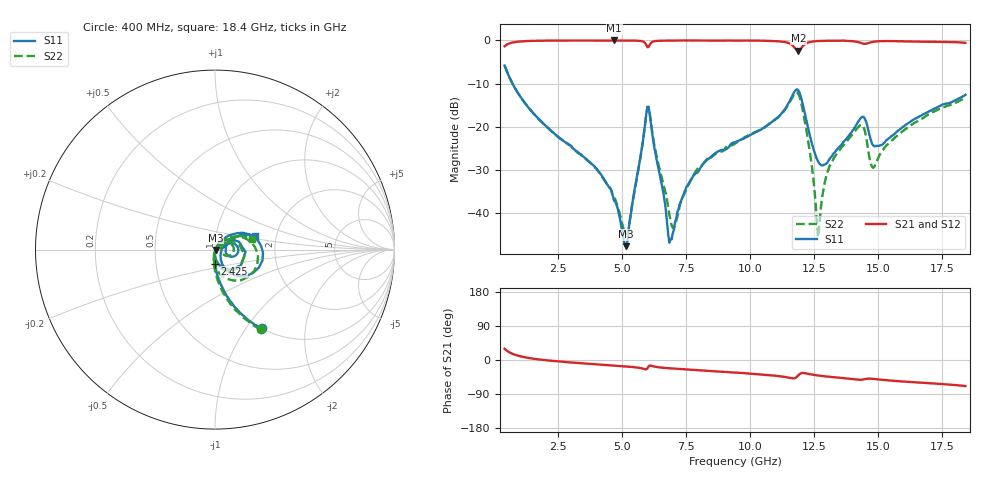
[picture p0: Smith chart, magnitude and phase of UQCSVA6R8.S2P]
!  Part Number  UQCSVA6R8  Mounting Orientation: Horizontal
!  Description: Ultra Low ESR Microwave capacitors
!  Application: Coupling, Bypass, Tuning, DC Block
!  Filters, Matching
# GHZ S DB R 50
! Freq  |S11|  S11 Ph  |S21|  S21 Ph  |S12|  S12 Ph  |S22|  S22 Ph
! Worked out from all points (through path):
!   401 points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, 400 MHz to 18.4 GHz, reference 50 ohm
!   highest |S21| = -0.01 dB at 4.675 GHz (marker M1); lowest = -2.4 dB at 11.88 GHz (marker M2)
!   group delay of S21, straight-line fit = 11.4 ps
!   lowest |S11| = -47.7 dB at 5.125 GHz (marker M3), VSWR 1.01, Z = 50.4 - j0.152 ohm
!   |S11| at or under -10 dB: 707.6 MHz to end of sweep
!   |S22| runs from -45.6 to -5.8 dB; largest |S21 - S12| = 0.0057
!   S11 on the Smith chart (normalised r, x): 400 MHz: 1.00, -1.19; 2.425 GHz: 0.98, -0.16; 18.4 GHz: 1.54, +0.25
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0.4  -5.83 -59.3  -1.37 29.6  -1.37 29.6  -5.82 -60.3
2.425  -22.00 -91.1  -0.04 -3.3  -0.05 -3.4  -22.05 -94.2
3.415  -26.57 -94.3  -0.03 -8.6  -0.03 -8.7  -26.70 -97.8
4.675  -37.14 -90.4  -0.01 -14.6  -0.01 -14.7  -36.35 -92.5
5.125  -47.67 -21.4  -0.03 -16.9  -0.03 -17.0  -44.82 -35.0
5.98  -15.38 -4.5  -1.56 -22.1  -1.54 -22.1  -15.44 -11.6
6.43  -30.29 -88.7  -0.08 -19.3  -0.09 -19.4  -29.18 -90.2
6.88  -45.96 -19.5  -0.05 -22.0  -0.04 -22.1  -41.56 -60.4
7.06  -41.97 28.9  -0.04 -22.9  -0.04 -23.0  -42.77 -2.9
7.735  -31.77 56.2  -0.02 -26.2  -0.04 -26.3  -31.75 44.7
9.4  -23.61 52.7  -0.06 -33.1  -0.07 -33.2  -23.92 48.6
11.425  -15.23 32.5  -0.47 -45.8  -0.47 -45.7  -15.42 23.2
11.875  -11.56 -22.4  -2.40 -40.6  -2.38 -40.5  -12.42 -39.1
12.415  -24.16 -58.5  -0.27 -38.5  -0.27 -38.6  -29.66 -98.5
12.595  -27.45 -43.1  -0.16 -40.5  -0.17 -40.5  -42.09 -73.0
12.685  -28.46 -32.7  -0.13 -41.3  -0.13 -41.3  -43.77 9.0
13.09  -27.51 9.0  -0.07 -44.3  -0.07 -44.3  -29.18 44.7
14.17  -19.27 17.8  -0.33 -51.6  -0.32 -51.6  -20.35 18.3
14.44  -17.83 -8.3  -0.79 -51.1  -0.79 -51.0  -20.35 -16.6
14.8  -24.32 -11.1  -0.31 -49.9  -0.32 -49.8  -29.52 3.7
15.43  -22.61 23.2  -0.15 -54.0  -0.15 -54.0  -23.70 34.3
18.4  -12.60 19.5  -0.57 -68.8  -0.53 -68.7  -13.30 15.2
